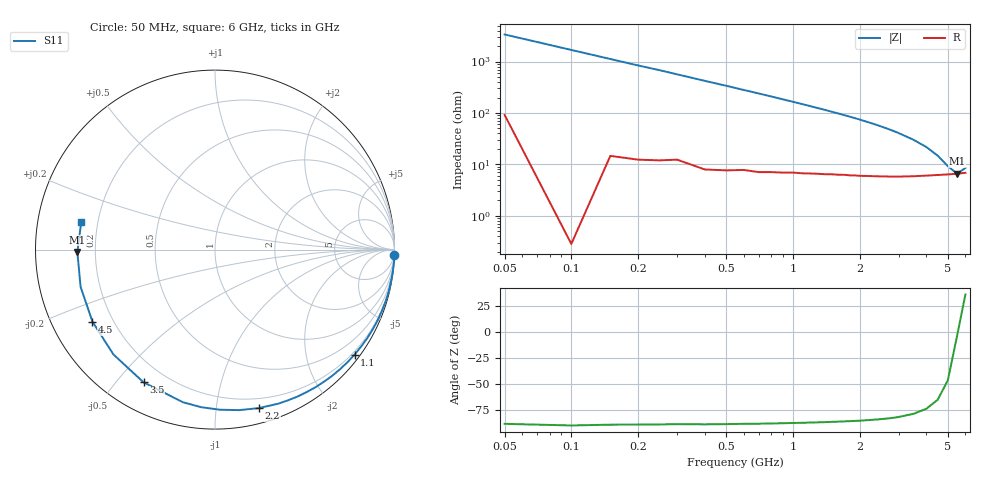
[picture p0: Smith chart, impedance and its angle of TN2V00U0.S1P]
! SIEMENS Discrete & RF Semiconductors
! BAS70-07W
! Si Schottky Diode in SOT343
! VR = 2 V
! S-Parameters:  February  1997
# GHz  S  MA  R  50
!  f  S11
! GHz  MAG  ANG
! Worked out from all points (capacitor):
!   34 points, 50 MHz to 6 GHz, reference 50 ohm
!   read as one part to ground: C = 945 fF near 50 MHz
!   lowest |Z| = 6.61 ohm at 5.5 GHz (marker M1)
!   series resonance near 5.539 GHz, so ESL is about 870 pH
!   S11 on the Smith chart (normalised r, x): 50 MHz: 2, -67; 1.1 GHz: 0.13, -2.98; 2.2 GHz: 0.12, -1.31; 3.5 GHz: 0.12, -0.59; 4.5 GHz: 0.12, -0.27; 6 GHz: 0.14, +0.10
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0.05  0.9992 -1.7
0.1  1 -3.4
0.2  0.9983 -6.8
0.4  0.9956 -13.5
0.5  0.9935 -16.8
0.6  0.9904 -20.2
0.7  0.9883 -23.5
0.8  0.9848 -26.9
0.9  0.9812 -30.3
1  0.977 -33.6
1.1  0.9733 -37.0
1.2  0.9687 -40.4
1.4  0.9595 -47.2
1.6  0.9493 -54.0
1.8  0.9389 -60.8
1.9  0.9331 -64.2
2  0.9282 -67.6
2.2  0.9162 -74.5
2.4  0.9045 -81.4
2.6  0.8926 -88.2
2.8  0.8813 -95.0
3  0.8691 -101.8
3.5  0.8398 -118.3
4  0.8134 -134.1
4.5  0.7921 -149.5
5  0.7771 -164.5
5.5  0.7669 -179.0
6  0.761 168.2
